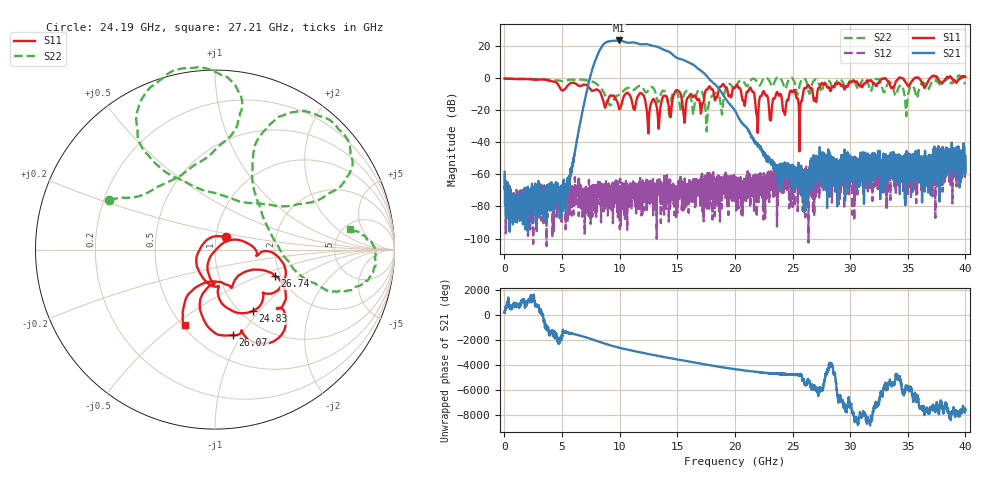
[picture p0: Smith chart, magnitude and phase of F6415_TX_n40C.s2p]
!Keysight Technologies,N5245B,MY52451815,A.15.70.20
!Date: Thursday, April 18, 2024 10:49:15
!Correction: S33(C  2-Port  )
!S43(C  2-Port  )
!S34(C  2-Port  )
!S44(C  2-Port  )
!S2P File: Measurements: S33, S43, S34, S44:
# Hz S  RI  R 50
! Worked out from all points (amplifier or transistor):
!   4000 points, 10 MHz to 40 GHz, reference 50 ohm
!   highest |S21| = 23.3 dB at 9.9 GHz (marker M1)
!   |S21| within 3 dB of that: 8.524 GHz to 12.69 GHz (4.162 GHz wide, 39.2 % of centre)
!   unconditionally stable (mu >= 1): start of sweep to 22.6 GHz; 24.94 GHz to 34.22 GHz; 34.41 GHz to 35.6 GHz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
!   at 6.67 GHz: K = 3482.44, MAG = -15.5 dB, |S12| = -69.9 dB
!   at 20.01 GHz: K = 21994.01, MAG = -18.4 dB, |S12| = -76.7 dB
!   at 40 GHz: K = -13399.29, MSG = -3.8 dB, |S12| = -50.7 dB
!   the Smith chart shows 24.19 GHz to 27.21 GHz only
!   S11 on the Smith chart (normalised r, x): 24.19 GHz: 1.12, +0.15; 24.83 GHz: 1.13, -0.92; 26.07 GHz: 0.74, -0.92; 26.74 GHz: 1.87, -0.63; 27.21 GHz: 0.51, -0.55
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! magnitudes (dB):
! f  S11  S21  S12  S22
! 10 MHz  -0.5  -58.4  -60.1  -0.4
! 750 MHz  -0.6  -75.9  -88.0  -0.5
! 4.86 GHz  -6.7  -70.8  -76.0  -1.8
! 6.68 GHz  -4.9  -23.8  -71.7  -1.0
! 8.22 GHz  -8.1  16.6  -71.9  -5.2
! 9.9 GHz  -18.0  23.3  -69.3  -10.6
! 11.87 GHz  -9.6  20.8  -69.7  -5.3
! 13.34 GHz  -27.6  19.2  -70.2  -15.1
! 14.97 GHz  -7.6  12.4  -70.9  -8.9
! 16.96 GHz  -16.2  4.9  -63.2  -7.4
! 17.57 GHz  -7.3  1.0  -81.4  -29.8
! 20.01 GHz  -5.9  -20.5  -76.7  -7.6
! 24.19 GHz  -20.8  -54.9  -65.4  -3.7
! 24.83 GHz  -7.9  -56.1  -60.4  0.2
! 25.66 GHz  -19.2  -61.2  -63.6  -3.2
! 26.07 GHz  -6.2  -58.3  -60.0  -0.6
! 26.67 GHz  -6.5  -52.4  -62.8  -4.4
! 26.74 GHz  -8.7  -52.5  -56.2  -2.9
! 27.21 GHz  -6.9  -56.5  -59.1  -2.3
! 33.34 GHz  -2.2  -63.6  -57.4  -2.9
! 34.87 GHz  -3.3  -68.6  -55.5  -23.8
! 40 GHz  0.7  -58.4  -50.7  -3.3
